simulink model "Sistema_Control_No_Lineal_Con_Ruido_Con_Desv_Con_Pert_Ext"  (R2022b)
settings: Solver=ode4  StartTime=0.0  StopTime=0.7  FixedStep=1e-6  RelTol=1e-3
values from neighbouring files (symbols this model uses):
  C_DC = 6.8e-3    (= 0.0068)    [Sistema_control_no_lineal_LQR.m]    (also in Sistema_control_no_lineal_Modal.m; PI_Lazo_V_DC.m; LQR_Sin_Integral.m; LQR_Con_Integral.m)
  control = eye(2)    [Sistema_control_no_lineal_LQR.m]    (also in Sistema_control_no_lineal_Modal.m; Sistema_no_lineal_Modal.m; Sistema_no_lineal_LQR.m)
  eta_d0_1 = ((i_q0_1*omega_1 + v_d_1/L_1 - (R_1/L_1)*i_d0_1)*(2*m_t1*L_1))/V_DC0    [Sistema_control_no_lineal_LQR.m]    (also in Sistema_control_no_lineal_Modal.m; Sistema_no_lineal_Modal.m; Sistema_no_lineal_LQR.m)
  eta_d0_2 = ((i_q0_2*omega_2 + v_d_2/L_2 - (R_2/L_2)*i_d0_2)*(2*m_t2*L_2))/V_DC0    [Sistema_control_no_lineal_LQR.m]    (also in Sistema_control_no_lineal_Modal.m; Sistema_no_lineal_Modal.m; Sistema_no_lineal_LQR.m)
  eta_q0_1 = (- i_d0_1*omega_1 - (R_1/L_1)*i_q0_1)*(2*m_t1*L_1)/V_DC0    [Sistema_control_no_lineal_LQR.m]    (also in Sistema_control_no_lineal_Modal.m; Sistema_no_lineal_Modal.m; Sistema_no_lineal_LQR.m)
  eta_q0_2 = ((- i_d0_2*omega_2 - (R_2/L_2)*i_q0_2)*(2*m_t2*L_2))/V_DC0    [Sistema_control_no_lineal_LQR.m]    (also in Sistema_control_no_lineal_Modal.m; Sistema_no_lineal_Modal.m; Sistema_no_lineal_LQR.m)
  i_d0_1 = ((3000*2)/(3*v_d_1))*1.06522    [Sistema_control_no_lineal_LQR.m]    (also in Sistema_control_no_lineal_Modal.m; PI_Lazo_V_DC.m = 14.14213562; Sistema_no_lineal_Modal.m; Sistema_no_lineal_LQR.m)
  i_d0_2 = -i_d0_1/1.06522    [Sistema_control_no_lineal_LQR.m]    (also in Sistema_control_no_lineal_Modal.m; Sistema_no_lineal_Modal.m; Sistema_no_lineal_LQR.m)
  I_p_i_d_1 = 0.2    [Sistema_control_no_lineal_LQR.m]    (also in Sistema_control_no_lineal_Modal.m; Sistema_no_lineal_Modal.m = 0.02; Sistema_no_lineal_LQR.m = 0.02)
  I_p_i_d_2 = 0.2    [Sistema_control_no_lineal_LQR.m]    (also in Sistema_control_no_lineal_Modal.m; Sistema_no_lineal_Modal.m = 0.02; Sistema_no_lineal_LQR.m = 0.02)
  I_p_i_q_1 = 0.2    [Sistema_control_no_lineal_LQR.m]    (also in Sistema_control_no_lineal_Modal.m; Sistema_no_lineal_Modal.m = 0.02; Sistema_no_lineal_LQR.m = 0.02)
  i_q0_1 = 0    [Sistema_control_no_lineal_LQR.m]    (also in Sistema_control_no_lineal_Modal.m; Sistema_no_lineal_Modal.m; Sistema_no_lineal_LQR.m)
  i_q0_2 = 0    [Sistema_control_no_lineal_LQR.m]    (also in Sistema_control_no_lineal_Modal.m; Sistema_no_lineal_Modal.m; Sistema_no_lineal_LQR.m)
  Inst_Desv_C_DC = 0.1    [Sistema_control_no_lineal_LQR.m]    (also in Sistema_control_no_lineal_Modal.m; Sistema_no_lineal_Modal.m; Sistema_no_lineal_LQR.m)
  Inst_Desv_L_1 = 0.1    [Sistema_control_no_lineal_LQR.m]    (also in Sistema_control_no_lineal_Modal.m; Sistema_no_lineal_Modal.m; Sistema_no_lineal_LQR.m)
  Inst_Desv_L_2 = 0.1    [Sistema_control_no_lineal_LQR.m]    (also in Sistema_control_no_lineal_Modal.m; Sistema_no_lineal_Modal.m; Sistema_no_lineal_LQR.m)
  Inst_Desv_R_1 = 0.1    [Sistema_control_no_lineal_LQR.m]    (also in Sistema_control_no_lineal_Modal.m; Sistema_no_lineal_Modal.m; Sistema_no_lineal_LQR.m)
  Inst_Desv_R_2 = 0.1    [Sistema_control_no_lineal_LQR.m]    (also in Sistema_control_no_lineal_Modal.m; Sistema_no_lineal_Modal.m; Sistema_no_lineal_LQR.m)
  Kc1 = Kca1(:, 1:2)    [Sistema_control_no_lineal_LQR.m]    (also in Sistema_control_no_lineal_Modal.m = Kca_place1(:, 1:2); Sistema_no_lineal_Modal.m = Kca_place1(:, 1:2); Sistema_no_lineal_LQR.m)
  Kc2 = Kca2(:, 1:2)    [Sistema_control_no_lineal_LQR.m]    (also in Sistema_control_no_lineal_Modal.m = Kca_place2(:, 1:2); Sistema_no_lineal_Modal.m = Kca_place2(:, 1:2); Sistema_no_lineal_LQR.m)
  Ki1 = -Kca1(:, 3:4)    [Sistema_control_no_lineal_LQR.m]    (also in Sistema_control_no_lineal_Modal.m = -Kca_place1(:, 3:4); Sistema_no_lineal_Modal.m = -Kca_place1(:, 3:4); Sistema_no_lineal_LQR.m)
  Ki2 = -Kca2(:, 3:4)    [Sistema_control_no_lineal_LQR.m]    (also in Sistema_control_no_lineal_Modal.m = -Kca_place2(:, 3:4); Sistema_no_lineal_Modal.m = -Kca_place2(:, 3:4); Sistema_no_lineal_LQR.m)
  Ki_DC = q_12/q_22    [Sistema_control_no_lineal_LQR.m]    (also in Sistema_control_no_lineal_Modal.m; PI_Lazo_V_DC.m)
  Ki_P = ((2+3*v_d_2*Kp_P)/(3*v_d_2*tau_P))    [Sistema_control_no_lineal_LQR.m]    (also in Sistema_control_no_lineal_Modal.m; IP_Lazo_P_2.m = ((2+3*v_d_2*Kp_P)/(3*v_d_2*tau)))
  Ki_Q = ((3*v_d_1*Kp_Q-2)/(3*v_d_1*tau_Q))    [Sistema_control_no_lineal_LQR.m]    (also in Sistema_control_no_lineal_Modal.m; IP_Lazo_Q_12.m = ((3*v_d_12*Kp_Q-2)/(3*v_d_12*tau)))
  Kp_DC = q_11/q_21    [Sistema_control_no_lineal_LQR.m]    (also in Sistema_control_no_lineal_Modal.m; PI_Lazo_V_DC.m)
  Kp_P = 0.0002    [Sistema_control_no_lineal_LQR.m]    (also in Sistema_control_no_lineal_Modal.m; IP_Lazo_P_2.m = 1)
  Kp_Q = 0.0002    [Sistema_control_no_lineal_LQR.m]    (also in Sistema_control_no_lineal_Modal.m; IP_Lazo_Q_12.m = 1)
  L_1 = 4.1e-3    (= 0.0041)    [Sistema_control_no_lineal_LQR.m]    (also in Sistema_control_no_lineal_Modal.m; Generadores_y_tranformadas.m; LQR_Sin_Integral.m; LQR_Con_Integral.m)
  L_2 = 5.3e-3    (= 0.0053)    [Sistema_control_no_lineal_LQR.m]    (also in Sistema_control_no_lineal_Modal.m; Generadores_y_tranformadas.m; Sistema_no_lineal_Modal.m; Sistema_no_lineal_LQR.m)
  lim_i_d_1_lower = -75.07117    [Sistema_control_no_lineal_LQR.m]    (also in Sistema_control_no_lineal_Modal.m; PI_Lazo_V_DC.m)
  lim_i_d_1_upper = 75.07117    [Sistema_control_no_lineal_LQR.m]    (also in Sistema_control_no_lineal_Modal.m; PI_Lazo_V_DC.m)
  lim_i_d_2_lower = -75.07117    [Sistema_control_no_lineal_LQR.m]    (also in Sistema_control_no_lineal_Modal.m; IP_Lazo_P_2.m)
  lim_i_d_2_upper = 75.07117    [Sistema_control_no_lineal_LQR.m]    (also in Sistema_control_no_lineal_Modal.m; IP_Lazo_P_2.m)
  lim_i_q_1_lower = -576.70686    [Sistema_control_no_lineal_LQR.m]    (also in Sistema_control_no_lineal_Modal.m; IP_Lazo_Q_12.m)
  lim_i_q_1_upper = 393.72177    [Sistema_control_no_lineal_LQR.m]    (also in Sistema_control_no_lineal_Modal.m; IP_Lazo_Q_12.m)
  m_t1 = 5    [Sistema_control_no_lineal_LQR.m]    (also in Sistema_control_no_lineal_Modal.m; LQR_Sin_Integral.m; LQR_Con_Integral.m; Modal_Integral.m)
  m_t2 = 5    [Sistema_control_no_lineal_LQR.m]    (also in Sistema_control_no_lineal_Modal.m; Sistema_no_lineal_Modal.m; Sistema_no_lineal_LQR.m)
  omega_1 = 377    [Sistema_control_no_lineal_LQR.m]    (also in Sistema_control_no_lineal_Modal.m; LQR_Sin_Integral.m; LQR_Con_Integral.m; Modal_Integral.m)
  omega_2 = 377    [Sistema_control_no_lineal_LQR.m]    (also in Sistema_control_no_lineal_Modal.m; Sistema_no_lineal_Modal.m; Sistema_no_lineal_LQR.m)
  P_2_1 = -3000    [Sistema_control_no_lineal_LQR.m]    (also in Sistema_control_no_lineal_Modal.m; IP_Lazo_P_2.m)
  P_2_2 = 3000    [Sistema_control_no_lineal_LQR.m]    (also in Sistema_control_no_lineal_Modal.m; IP_Lazo_P_2.m)
  P_2_3 = -8000    [Sistema_control_no_lineal_LQR.m]    (also in Sistema_control_no_lineal_Modal.m)
  p_i_d_1 = 2.5    [Sistema_control_no_lineal_LQR.m]    (also in Sistema_control_no_lineal_Modal.m; Sistema_no_lineal_Modal.m = 1.5; Sistema_no_lineal_LQR.m = 1.5)
  p_i_d_2 = 2.7    [Sistema_control_no_lineal_LQR.m]    (also in Sistema_control_no_lineal_Modal.m; Sistema_no_lineal_Modal.m = 1.7; Sistema_no_lineal_LQR.m = 1.7)
  p_i_q_1 = -0.5    [Sistema_control_no_lineal_LQR.m]    (also in Sistema_control_no_lineal_Modal.m; Sistema_no_lineal_Modal.m = -1.3; Sistema_no_lineal_LQR.m = -1.3)
  Porc_Desv_C_DC = 0.05    [Sistema_control_no_lineal_LQR.m]    (also in Sistema_control_no_lineal_Modal.m; Sistema_no_lineal_Modal.m; Sistema_no_lineal_LQR.m)
  Porc_Desv_L_1 = 0.05    [Sistema_control_no_lineal_LQR.m]    (also in Sistema_control_no_lineal_Modal.m; Sistema_no_lineal_Modal.m; Sistema_no_lineal_LQR.m)
  Porc_Desv_L_2 = 0.05    [Sistema_control_no_lineal_LQR.m]    (also in Sistema_control_no_lineal_Modal.m; Sistema_no_lineal_Modal.m; Sistema_no_lineal_LQR.m)
  Porc_Desv_R_1 = 0.05    [Sistema_control_no_lineal_LQR.m]    (also in Sistema_control_no_lineal_Modal.m; Sistema_no_lineal_Modal.m; Sistema_no_lineal_LQR.m)
  Porc_Desv_R_2 = 0.05    [Sistema_control_no_lineal_LQR.m]    (also in Sistema_control_no_lineal_Modal.m; Sistema_no_lineal_Modal.m; Sistema_no_lineal_LQR.m)
  Q_1_1 = 0    [Sistema_control_no_lineal_LQR.m]    (also in Sistema_control_no_lineal_Modal.m; IP_Lazo_Q_12.m)
  Q_1_2 = 0    [Sistema_control_no_lineal_LQR.m]    (also in Sistema_control_no_lineal_Modal.m; IP_Lazo_Q_12.m = -2500)
  Q_1_3 = 0    [Sistema_control_no_lineal_LQR.m]    (also in Sistema_control_no_lineal_Modal.m)
  Q_2_1 = 0    [Sistema_control_no_lineal_LQR.m]    (also in Sistema_control_no_lineal_Modal.m; IP_Lazo_Q_12.m = -3000)
  Q_2_2 = 0    [Sistema_control_no_lineal_LQR.m]    (also in Sistema_control_no_lineal_Modal.m; IP_Lazo_Q_12.m = 1000)
  Q_2_3 = 0    [Sistema_control_no_lineal_LQR.m]    (also in Sistema_control_no_lineal_Modal.m)
  R_1 = 284e-3    (= 0.284)    [Sistema_control_no_lineal_LQR.m]    (also in Sistema_control_no_lineal_Modal.m; Generadores_y_tranformadas.m; LQR_Sin_Integral.m; LQR_Con_Integral.m)
  R_2 = 330e-3    (= 0.33)    [Sistema_control_no_lineal_LQR.m]    (also in Sistema_control_no_lineal_Modal.m; Generadores_y_tranformadas.m; Sistema_no_lineal_Modal.m; Sistema_no_lineal_LQR.m)
  v_d_1 = 100*sqrt(2)    [Sistema_control_no_lineal_LQR.m]    (also in Sistema_control_no_lineal_Modal.m; PI_Lazo_V_DC.m; LQR_Sin_Integral.m; LQR_Con_Integral.m)
  v_d_2 = 100*sqrt(2)    [Sistema_control_no_lineal_LQR.m]    (also in Sistema_control_no_lineal_Modal.m; IP_Lazo_P_2.m; Sistema_no_lineal_Modal.m; Sistema_no_lineal_LQR.m)
  V_DC0 = 500    [Sistema_control_no_lineal_LQR.m]    (also in Sistema_control_no_lineal_Modal.m; PI_Lazo_V_DC.m; LQR_Sin_Integral.m; LQR_Con_Integral.m)
  V_R_C = D_R_V^2    (= 0.0009)    [Sistema_control_no_lineal_LQR.m]    (also in Sistema_control_no_lineal_Modal.m)
  V_R_i = D_R_i^2    (= 2.5e-05)    [Sistema_control_no_lineal_LQR.m]    (also in Sistema_control_no_lineal_Modal.m; LQR_Con_Integral.m; Modal_Integral.m; Sistema_no_lineal_Modal.m)
  V_R_V = D_R_V^2    (= 0.0009)    [Sistema_control_no_lineal_LQR.m]    (also in Sistema_control_no_lineal_Modal.m; PI_Lazo_V_DC.m; Sistema_no_lineal_Modal.m = 4e-06; Sistema_no_lineal_LQR.m = 4e-06)

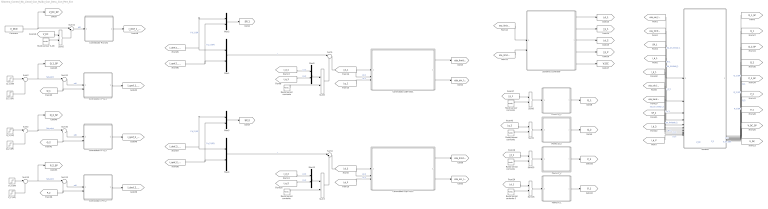
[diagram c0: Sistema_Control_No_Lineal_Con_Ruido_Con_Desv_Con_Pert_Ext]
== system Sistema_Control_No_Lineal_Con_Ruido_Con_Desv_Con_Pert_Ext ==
  "   Ruido sensor corriente " : RandomNumber  Variance=V_R_i  SampleTime=0.001
  "   Ruido sensor corriente 1" : RandomNumber  Variance=V_R_i  SampleTime=0.001
  "  Ruido sensor corriente " : RandomNumber  Variance=V_R_i  SampleTime=0.001
  " Ruido sensor corriente " : RandomNumber  Variance=V_R_i  SampleTime=0.001
  Constant : Constant  Value=V_DC0
  Controlador I-P P_2 : Subsystem
  Controlador I-P Q_1 : Subsystem
  Controlador I-P Q_2 : Subsystem
  Controlador LQR VSC1 : Subsystem
  Controlador LQR VSC2 : Subsystem
  Controlador PI V_DC : Subsystem
  Mux{1..2,4..5,9,12} (6 alike) : Mux  Inputs=2
  P_2 (SP) : Step  Time=0.3  Before=P_2_1  After=P_2_2  SampleTime=0
  "P_2 (SP) " : Step  Time=0.5  After=P_2_3  SampleTime=0
  Planta P_1 : Subsystem
  Planta P_2 : Subsystem
  Planta Q_1 : Subsystem
  Planta Q_2 : Subsystem
  Q_1 (SP) : Step  Time=0.3  Before=Q_1_1  After=Q_1_2  SampleTime=0
  "Q_1 (SP) " : Step  Time=0.5  After=Q_1_3  SampleTime=0
  Q_2 (SP) : Step  Time=0.4  Before=Q_2_1  After=Q_2_2  SampleTime=0
  "Q_2 (SP) " : Step  Time=0.5  After=Q_2_3  SampleTime=0
  Ruido sensor V_DC : RandomNumber  Variance=V_R_V  SampleTime=0.001
  Ruido sensor corriente : RandomNumber  Variance=V_R_i  SampleTime=0.001
  "Ruido sensor corriente " : RandomNumber  Variance=V_R_i  SampleTime=0.001
  Señales : Subsystem
  Sistema a controlar : Subsystem
  Sum{1,4,10..13} (6 alike) : Sum  Inputs=|+-
  Sum14 : Sum  Inputs=|++
  Sum{5..9,15..16} (7 alike) : Sum
  Sum2 : Sum  Inputs=|++
  Sum3 : Sum  Inputs=|++
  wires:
  Mux2/1 -> [SP_1]
  [i_dref_1_limitado] -> Mux2/1, Mux1/1  "i^d_1 (SP)"
  [i_qref_1_limitado] -> Mux2/2, Mux1/2  "i^q_1 (SP)"
  Mux1/1 -> Sum1/1  "r"
  [i_qref_2_limitado] -> Mux5/2, Mux4/2  "i^q_2 (SP)"
  [i_dref_2_limitado] -> Mux4/1, Mux5/1  "i^d_2 (SP)"
  Mux5/1 -> [SP_2]
  Sistema a controlar/1(i_d_1) -> [i_d_1]
  Sistema a controlar/2(i_q_1) -> [i_q_1]
  Sistema a controlar/3(i_d_2) -> [i_d_2]
  Sistema a controlar/4(i_q_2) -> [i_q_2]
  Sistema a controlar/5(V_DC) -> [V_DC]
  [eta_limitado_1] -> Sistema a controlar/1(eta limitado 1)
  [eta_limitado_2] -> Sistema a controlar/2(eta limitado 2)
  [i_d_1] -> Mux9/1  "i_d_2"
  [i_q_1] -> Mux9/2  "i_q_2"
  Sum6/1 -> Sum1/2
  Sum7/1 -> Sum4/2
  [i_q_2] -> Mux12/2  "i_q_2"
  [i_d_2] -> Mux12/1  "i_d_2"
  Mux4/1 -> Sum4/1  "r"
  Sum1/1 -> Controlador LQR VSC1/1(e)
  [i_d_1] -> Controlador LQR VSC1/2(i_d_1)  "i_d_1"
  [i_q_1] -> Controlador LQR VSC1/3(i_q_1)  "i_q_1"
  Controlador LQR VSC1/1(eta limitado 1) -> [eta_limitado_1]
  Controlador LQR VSC1/2(eta sin limitar 1) -> [eta_sin_limitar_1]
  Sum4/1 -> Controlador LQR VSC2/1(e)
  [i_d_2] -> Controlador LQR VSC2/2(i_d_2)  "i_d_2"
  [i_q_2] -> Controlador LQR VSC2/3(i_q_2)  "i_q_2"
  Controlador LQR VSC2/1(eta limitado 2) -> [eta_limitado_2]
  Controlador LQR VSC2/2(eta sin limitar 2) -> [eta_sin_limitar_2]
  Controlador I-P Q_1/1(i^q*_1 limitado) -> [i_qref_1_limitado]
  Sum12/1 -> Controlador I-P Q_1/1(e(t))  "e(t)"
  P_2 (SP)/1 -> Sum14/1
  Sum3/1 -> [Q_1_SP], Sum12/1  "Set-point"
  Controlador PI V_DC/1(i^d*_1 limitado) -> [i_dref_1_limitado]
  Sum13/1 -> Controlador I-P P_2/1(e(t))  "e(t)"
  Sum11/1 -> Controlador PI V_DC/1(e(t))  "e(t)"
  "P_2 (SP) "/1 -> Sum14/2
  Sum5/1 -> Sum11/2
  Controlador I-P P_2/1(i^d*_2 limitado) -> [i_dref_2_limitado]
  Sum10/1 -> Controlador I-P Q_2/1(e(t))  "e(t)"
  [P_2] -> Controlador I-P P_2/2(P_2), Sum13/2
  [Q_1] -> Controlador I-P Q_1/2(Q_1), Sum12/2
  [Q_2] -> Sum10/2, Controlador I-P Q_2/2(Q_1)
  Controlador I-P Q_2/1(i^q*_1 limitado) -> [i_qref_2_limitado]
  Sum2/1 -> Sum10/1, [Q_2_SP]  "Set-point"
  Sum14/1 -> [P_2_SP], Sum13/1  "Set-point"
  Constant/1 -> [V_DC_SP], Sum11/1
  Q_2 (SP)/1 -> Sum2/1
  "Q_2 (SP) "/1 -> Sum2/2
  Q_1 (SP)/1 -> Sum3/1
  "Q_1 (SP) "/1 -> Sum3/2
  [V_DC] -> Sum5/1
  Ruido sensor V_DC/1 -> Sum5/2
  Mux9/1 -> Sum6/1
  Ruido sensor corriente/1 -> Sum6/2
  Mux12/1 -> Sum7/1
  "Ruido sensor corriente "/1 -> Sum7/2
  [V_DC_SP] -> Señales/18(V_DC (SP))  "V_DC (SP)"
  [eta_limitado_1] -> Señales/2(eta_limitado_1)  "eta_limitado_1"
  [P_2] -> Señales/16(P_2)  "P_2"
  [i_q_1] -> Señales/5(i_q_1)  "i_q_1"
  [i_d_2] -> Señales/9(i_d_2)  "i_d_1"
  [i_q_2] -> Señales/10(i_q_2)  "i_q_1"
  [eta_sin_limitar_2] -> Señales/6(eta_sin_limitar_2)  "eta_sin_limitar_2"
  [Q_1] -> Señales/12(Q_1)  "Q_1"
  [eta_sin_limitar_1] -> Señales/1(eta_sin_limitar_1)  "eta_sin_limitar_1"
  [SP_2] -> Señales/8(SP_2)  "SP_2"
  [Q_1_SP] -> Señales/11(Q_1 (SP))  "Q_1 (SP)"
  [eta_limitado_2] -> Señales/7(eta_limitado_2)  "eta_limitado_2"
  [i_d_1] -> Señales/4(i_d_1)  "i_d_1"
  [P_2_SP] -> Señales/15(P_2 (SP))  "P_2 (SP)"
  [Q_2_SP] -> Señales/13(Q_2 (SP))  "Q_2 (SP)"
  [SP_1] -> Señales/3(SP_1)  "SP_1"
  [Q_2] -> Señales/14(Q_2)  "Q_2"
  [P_1] -> Señales/17(P_1)  "P_1"
  [V_DC] -> Señales/19(V_DC)  "V_DC"
  [i_q_2] -> Sum9/1
  Planta P_2/1(P_2) -> [P_2]
  [i_d_2] -> Sum15/1
  Planta Q_2/1(Q_2) -> [Q_2]
  "  Ruido sensor corriente "/1 -> Sum9/2
  [i_d_1] -> Sum16/1
  Sum16/1 -> Planta P_1/1(i^d*_1 limitado)
  Planta P_1/1(P_1) -> [P_1]
  Planta Q_1/1(Q_1) -> [Q_1]
  [i_q_1] -> Sum8/1
  " Ruido sensor corriente "/1 -> Sum8/2
  Sum8/1 -> Planta Q_1/1(i^q*_1 limitado)
  "   Ruido sensor corriente "/1 -> Sum15/2
  Sum9/1 -> Planta Q_2/1(i^q*_2 limitado)
  Sum15/1 -> Planta P_2/1(i^d*_2 limitado)
  "   Ruido sensor corriente 1"/1 -> Sum16/2

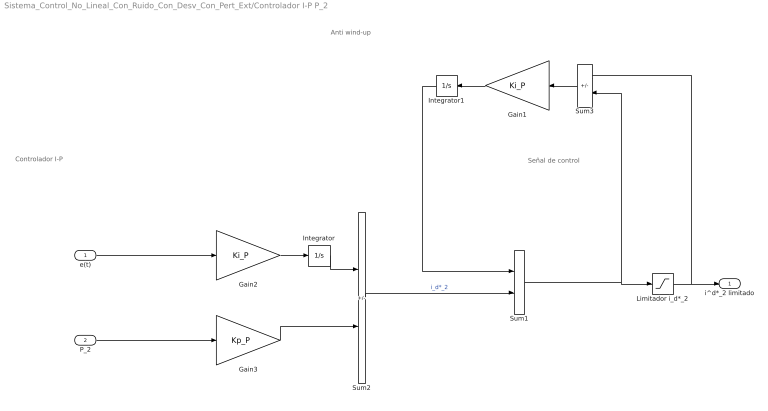
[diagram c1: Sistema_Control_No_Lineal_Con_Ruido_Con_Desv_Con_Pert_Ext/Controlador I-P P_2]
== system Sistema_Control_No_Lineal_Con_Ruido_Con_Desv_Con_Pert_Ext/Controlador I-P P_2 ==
  note: Señal de control
  note: Controlador I-P
  note: Anti wind-up
  e(t) : Inport
  P_2 : Inport  Port=2
  Gain1 : Gain  Gain=Ki_P
  Gain2 : Gain  Gain=Ki_P
  Gain3 : Gain  Gain=Kp_P
  Integrator : Integrator
  Integrator1 : Integrator
  Limitador i_d*_2 : Saturate  UpperLimit=lim_i_d_2_upper  LowerLimit=lim_i_d_2_lower
  Sum1 : Sum
  Sum2 : Sum  Inputs=+-
  Sum3 : Sum  Inputs=+-
  i^d*_2 limitado : Outport
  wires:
  Limitador i_d*_2/1 -> i^d*_2 limitado/1, Sum3/1
  Sum1/1 -> Limitador i_d*_2/1, Sum3/2
  Sum2/1 -> Sum1/2  "i_d*_2"
  Gain2/1 -> Integrator/1
  Integrator/1 -> Sum2/1
  e(t)/1 -> Gain2/1
  Sum3/1 -> Gain1/1
  Gain1/1 -> Integrator1/1
  Integrator1/1 -> Sum1/1
  P_2/1 -> Gain3/1
  Gain3/1 -> Sum2/2

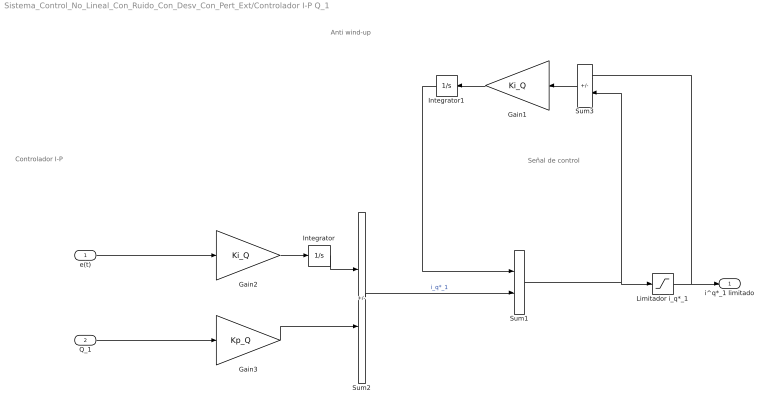
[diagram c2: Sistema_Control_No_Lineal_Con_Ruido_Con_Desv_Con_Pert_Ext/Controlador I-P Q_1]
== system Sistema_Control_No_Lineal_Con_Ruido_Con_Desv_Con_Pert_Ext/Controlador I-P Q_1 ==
  note: Señal de control
  note: Controlador I-P
  note: Anti wind-up
  e(t) : Inport
  Q_1 : Inport  Port=2
  Gain1 : Gain  Gain=Ki_Q
  Gain2 : Gain  Gain=Ki_Q
  Gain3 : Gain  Gain=Kp_Q
  Integrator : Integrator
  Integrator1 : Integrator
  Limitador i_q*_1 : Saturate  UpperLimit=lim_i_q_1_upper  LowerLimit=lim_i_q_1_lower
  Sum1 : Sum
  Sum2 : Sum  Inputs=+-
  Sum3 : Sum  Inputs=+-
  i^q*_1 limitado : Outport
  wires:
  Limitador i_q*_1/1 -> i^q*_1 limitado/1, Sum3/1
  Sum1/1 -> Limitador i_q*_1/1, Sum3/2
  Sum2/1 -> Sum1/2  "i_q*_1"
  Gain2/1 -> Integrator/1
  Integrator/1 -> Sum2/1
  e(t)/1 -> Gain2/1
  Sum3/1 -> Gain1/1
  Gain1/1 -> Integrator1/1
  Integrator1/1 -> Sum1/1
  Q_1/1 -> Gain3/1
  Gain3/1 -> Sum2/2

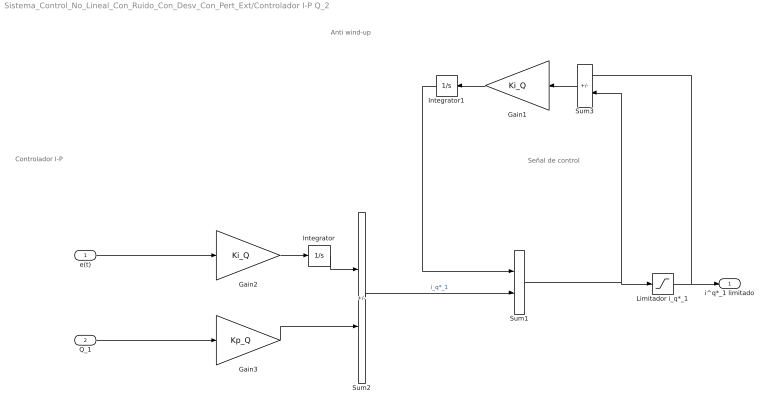
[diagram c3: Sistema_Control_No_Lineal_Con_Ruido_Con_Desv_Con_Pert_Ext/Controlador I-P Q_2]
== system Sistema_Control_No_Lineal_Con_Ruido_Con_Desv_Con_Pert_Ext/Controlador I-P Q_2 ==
  note: Anti wind-up
  note: Controlador I-P
  note: Señal de control
  e(t) : Inport
  Q_1 : Inport  Port=2
  Gain1 : Gain  Gain=Ki_Q
  Gain2 : Gain  Gain=Ki_Q
  Gain3 : Gain  Gain=Kp_Q
  Integrator : Integrator
  Integrator1 : Integrator
  Limitador i_q*_1 : Saturate  UpperLimit=lim_i_q_1_upper  LowerLimit=lim_i_q_1_lower
  Sum1 : Sum
  Sum2 : Sum  Inputs=+-
  Sum3 : Sum  Inputs=+-
  i^q*_1 limitado : Outport
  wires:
  Gain3/1 -> Sum2/2
  Q_1/1 -> Gain3/1
  Integrator1/1 -> Sum1/1
  Gain1/1 -> Integrator1/1
  Sum3/1 -> Gain1/1
  e(t)/1 -> Gain2/1
  Integrator/1 -> Sum2/1
  Gain2/1 -> Integrator/1
  Sum2/1 -> Sum1/2  "i_q*_1"
  Sum1/1 -> Sum3/2, Limitador i_q*_1/1
  Limitador i_q*_1/1 -> Sum3/1, i^q*_1 limitado/1

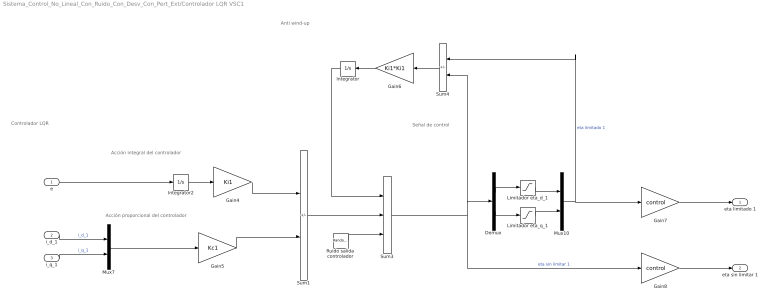
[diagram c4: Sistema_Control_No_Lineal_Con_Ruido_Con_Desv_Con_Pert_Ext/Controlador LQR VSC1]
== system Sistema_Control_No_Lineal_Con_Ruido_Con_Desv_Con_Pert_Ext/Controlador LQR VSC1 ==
  note: Anti wind-up
  note: Controlador LQR
  note: Acción proporcional del controlador
  note: Acción integral del controlador
  note: Señal de control
  e : Inport
  i_d_1 : Inport  Port=2
  i_q_1 : Inport  Port=3
  Demux : Demux  Outputs=2
  Gain4 : Gain  Gain=Ki1  Multiplication=Matrix(K*u) (u vector)
  Gain5 : Gain  Gain=Kc1  Multiplication=Matrix(K*u) (u vector)
  Gain6 : Gain  Gain=Ki1*Ki1  Multiplication=Matrix(K*u) (u vector)
  Gain7 : Gain  Gain=control  Multiplication=Matrix(K*u) (u vector)
  Gain8 : Gain  Gain=control  Multiplication=Matrix(K*u) (u vector)
  Integrator : Integrator
  Integrator2 : Integrator
  Limitador eta_d_1 : Saturate  UpperLimit=5 - eta_d0_1  LowerLimit=-5 - eta_d0_1
  Limitador eta_q_1 : Saturate  UpperLimit=5 - eta_q0_1  LowerLimit=-5 - eta_q0_1
  Mux10 : Mux  Inputs=2
  Mux7 : Mux  Inputs=2
  Ruido salida controlador : RandomNumber  Variance=V_R_C  SampleTime=0.001
  Sum1 : Sum  Inputs=+-
  Sum3 : Sum  Inputs=+++
  Sum4 : Sum  Inputs=+-
  eta limitado 1 : Outport
  eta sin limitar 1 : Outport  Port=2
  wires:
  i_q_1/1 -> Mux7/2  "i_q_1"
  Mux10/1 -> Sum4/1, Gain7/1  "eta limitado 1"
  Limitador eta_q_1/1 -> Mux10/2
  i_d_1/1 -> Mux7/1  "i_d_1"
  Limitador eta_d_1/1 -> Mux10/1
  Demux/2 -> Limitador eta_q_1/1
  Gain8/1 -> eta sin limitar 1/1
  Sum3/1 -> Demux/1, Sum4/2, Gain8/1  "eta sin limitar 1"
  Gain7/1 -> eta limitado 1/1
  Demux/1 -> Limitador eta_d_1/1
  Gain5/1 -> Sum1/2
  Gain4/1 -> Sum1/1
  Sum4/1 -> Gain6/1
  Mux7/1 -> Gain5/1
  Gain6/1 -> Integrator/1
  Sum1/1 -> Sum3/2
  Integrator2/1 -> Gain4/1
  e/1 -> Integrator2/1
  Integrator/1 -> Sum3/1
  Ruido salida controlador/1 -> Sum3/3

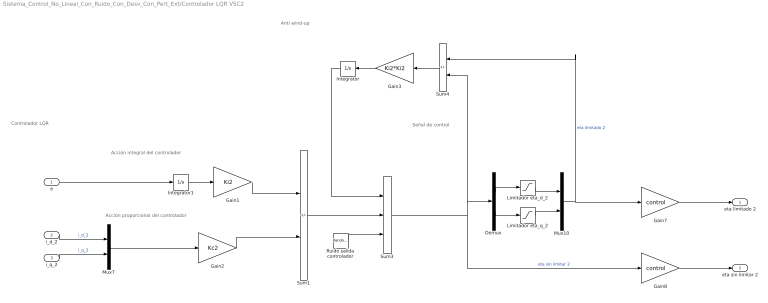
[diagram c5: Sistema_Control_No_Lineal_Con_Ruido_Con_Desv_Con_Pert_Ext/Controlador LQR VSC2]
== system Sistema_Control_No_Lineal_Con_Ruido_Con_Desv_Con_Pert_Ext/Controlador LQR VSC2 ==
  note: Señal de control
  note: Anti wind-up
  note: Acción proporcional del controlador
  note: Controlador LQR
  note: Acción integral del controlador
  e : Inport
  i_d_2 : Inport  Port=2
  i_q_2 : Inport  Port=3
  Demux : Demux  Outputs=2
  Gain1 : Gain  Gain=Ki2  Multiplication=Matrix(K*u) (u vector)
  Gain2 : Gain  Gain=Kc2  Multiplication=Matrix(K*u) (u vector)
  Gain3 : Gain  Gain=Ki2*Ki2  Multiplication=Matrix(K*u) (u vector)
  Gain7 : Gain  Gain=control  Multiplication=Matrix(K*u) (u vector)
  Gain8 : Gain  Gain=control  Multiplication=Matrix(K*u) (u vector)
  Integrator : Integrator
  Integrator1 : Integrator
  Limitador eta_d_2 : Saturate  UpperLimit=5 - eta_d0_2  LowerLimit=-5 - eta_d0_2
  Limitador eta_q_2 : Saturate  UpperLimit=5 - eta_q0_2  LowerLimit=-5 - eta_q0_2
  Mux10 : Mux  Inputs=2
  Mux7 : Mux  Inputs=2
  Ruido salida controlador : RandomNumber  Variance=V_R_C  SampleTime=0.001
  Sum1 : Sum  Inputs=+-
  Sum3 : Sum  Inputs=+++
  Sum4 : Sum  Inputs=+-
  eta limitado 2 : Outport
  eta sin limitar 2 : Outport  Port=2
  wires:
  Gain8/1 -> eta sin limitar 2/1
  Integrator/1 -> Sum3/1
  Mux7/1 -> Gain2/1
  i_d_2/1 -> Mux7/1  "i_d_2"
  Mux10/1 -> Sum4/1, Gain7/1  "eta limitado 2"
  Gain7/1 -> eta limitado 2/1
  Sum3/1 -> Demux/1, Sum4/2, Gain8/1  "eta sin limitar 2"
  i_q_2/1 -> Mux7/2  "i_q_2"
  Limitador eta_d_2/1 -> Mux10/1
  Limitador eta_q_2/1 -> Mux10/2
  Integrator1/1 -> Gain1/1
  Demux/2 -> Limitador eta_q_2/1
  Demux/1 -> Limitador eta_d_2/1
  Sum4/1 -> Gain3/1
  Gain3/1 -> Integrator/1
  Sum1/1 -> Sum3/2
  Gain1/1 -> Sum1/1
  Gain2/1 -> Sum1/2
  e/1 -> Integrator1/1
  Ruido salida controlador/1 -> Sum3/3

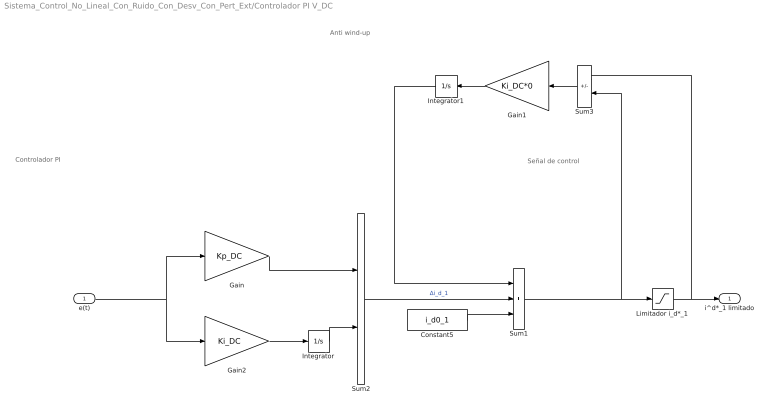
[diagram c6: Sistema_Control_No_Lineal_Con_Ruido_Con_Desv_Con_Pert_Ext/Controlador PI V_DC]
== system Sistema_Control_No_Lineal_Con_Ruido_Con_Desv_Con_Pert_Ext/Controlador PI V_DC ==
  note: Señal de control
  note: Controlador PI
  note: Anti wind-up
  e(t) : Inport
  Constant5 : Constant  Value=i_d0_1
  Gain : Gain  Gain=Kp_DC
  Gain1 : Gain  Gain=Ki_DC*0
  Gain2 : Gain  Gain=Ki_DC
  Integrator : Integrator
  Integrator1 : Integrator
  Limitador i_d*_1 : Saturate  UpperLimit=lim_i_d_1_upper  LowerLimit=lim_i_d_1_lower
  Sum1 : Sum  Inputs=+++
  Sum2 : Sum
  Sum3 : Sum  Inputs=+-
  i^d*_1 limitado : Outport
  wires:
  Limitador i_d*_1/1 -> Sum3/1, i^d*_1 limitado/1
  Constant5/1 -> Sum1/3
  Sum1/1 -> Sum3/2, Limitador i_d*_1/1
  Sum2/1 -> Sum1/2  "Δi_d_1"
  Gain2/1 -> Integrator/1
  Integrator/1 -> Sum2/2
  Gain/1 -> Sum2/1
  e(t)/1 -> Gain2/1, Gain/1
  Sum3/1 -> Gain1/1
  Gain1/1 -> Integrator1/1
  Integrator1/1 -> Sum1/1

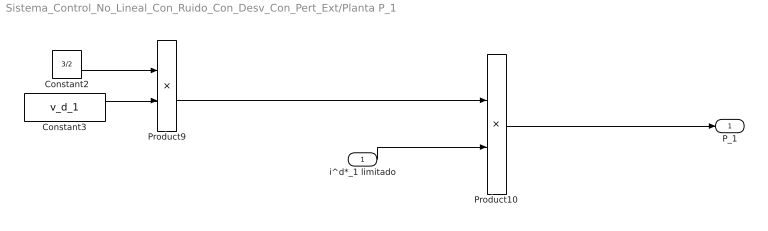
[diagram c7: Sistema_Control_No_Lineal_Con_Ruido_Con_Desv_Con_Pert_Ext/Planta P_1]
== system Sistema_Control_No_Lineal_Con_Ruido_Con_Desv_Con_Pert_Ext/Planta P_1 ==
  i^d*_1 limitado : Inport
  Constant2 : Constant  Value=3/2
  Constant3 : Constant  Value=v_d_1
  Product10 : Product
  Product9 : Product
  P_1 : Outport
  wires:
  Product10/1 -> P_1/1
  Constant2/1 -> Product9/1
  Constant3/1 -> Product9/2
  i^d*_1 limitado/1 -> Product10/2
  Product9/1 -> Product10/1

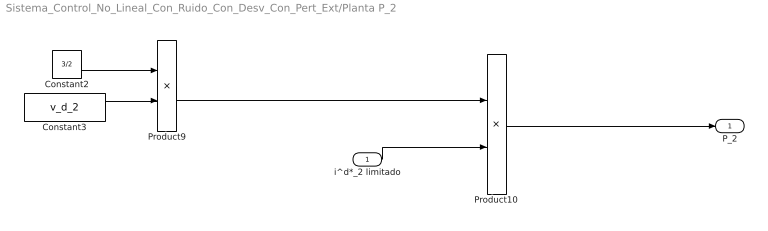
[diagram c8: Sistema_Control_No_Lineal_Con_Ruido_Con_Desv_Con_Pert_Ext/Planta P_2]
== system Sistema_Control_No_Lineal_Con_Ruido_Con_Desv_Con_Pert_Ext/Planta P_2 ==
  i^d*_2 limitado : Inport
  Constant2 : Constant  Value=3/2
  Constant3 : Constant  Value=v_d_2
  Product10 : Product
  Product9 : Product
  P_2 : Outport
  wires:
  Product9/1 -> Product10/1
  i^d*_2 limitado/1 -> Product10/2
  Constant3/1 -> Product9/2
  Constant2/1 -> Product9/1
  Product10/1 -> P_2/1

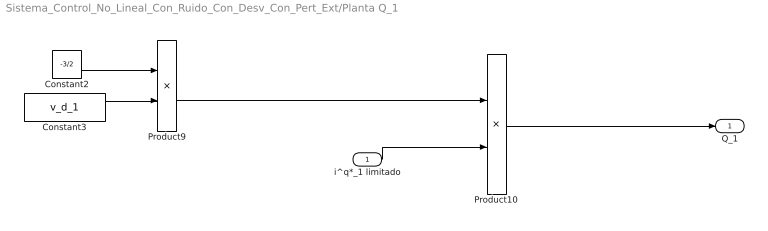
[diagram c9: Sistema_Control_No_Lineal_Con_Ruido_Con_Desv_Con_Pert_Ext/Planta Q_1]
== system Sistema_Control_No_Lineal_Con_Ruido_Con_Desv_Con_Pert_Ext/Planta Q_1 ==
  i^q*_1 limitado : Inport
  Constant2 : Constant  Value=-3/2
  Constant3 : Constant  Value=v_d_1
  Product10 : Product
  Product9 : Product
  Q_1 : Outport
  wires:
  Constant2/1 -> Product9/1
  Constant3/1 -> Product9/2
  i^q*_1 limitado/1 -> Product10/2
  Product9/1 -> Product10/1
  Product10/1 -> Q_1/1

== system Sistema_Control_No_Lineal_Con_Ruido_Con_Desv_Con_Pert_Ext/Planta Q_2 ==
  i^q*_2 limitado : Inport
  Constant2 : Constant  Value=-3/2
  Constant3 : Constant  Value=v_d_2
  Product10 : Product
  Product9 : Product
  Q_2 : Outport
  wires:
  Product9/1 -> Product10/1
  i^q*_2 limitado/1 -> Product10/2
  Constant3/1 -> Product9/2
  Constant2/1 -> Product9/1
  Product10/1 -> Q_2/1

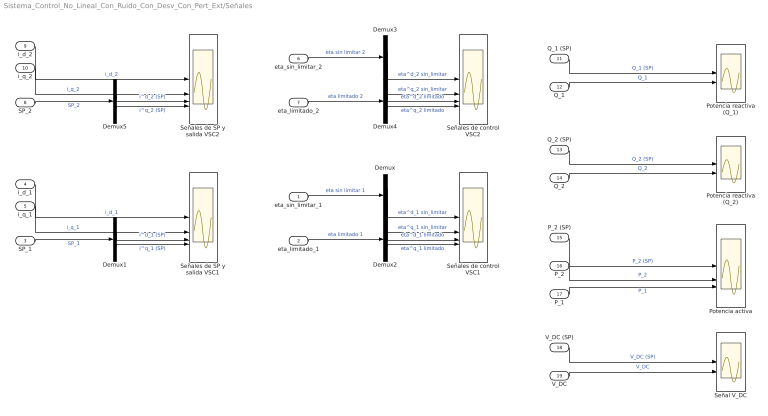
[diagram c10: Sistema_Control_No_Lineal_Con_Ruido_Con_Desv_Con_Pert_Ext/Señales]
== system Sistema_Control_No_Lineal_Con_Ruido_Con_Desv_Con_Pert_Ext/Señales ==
  eta_sin_limitar_1 : Inport
  eta_limitado_1 : Inport  Port=2
  SP_1 : Inport  Port=3
  i_d_1 : Inport  Port=4
  i_q_1 : Inport  Port=5
  eta_sin_limitar_2 : Inport  Port=6
  eta_limitado_2 : Inport  Port=7
  SP_2 : Inport  Port=8
  i_d_2 : Inport  Port=9
  i_q_2 : Inport  Port=10
  Q_1 (SP) : Inport  Port=11
  Q_1 : Inport  Port=12
  Q_2 (SP) : Inport  Port=13
  Q_2 : Inport  Port=14
  P_2 (SP) : Inport  Port=15
  P_2 : Inport  Port=16
  P_1 : Inport  Port=17
  V_DC (SP) : Inport  Port=18
  V_DC : Inport  Port=19
  Demux{,1..5} (6 alike) : Demux  Outputs=2
  Potencia activa : Scope  NumInputPorts=3
  Potencia reactiva (Q_1) : Scope  NumInputPorts=2
  Potencia reactiva (Q_2) : Scope  NumInputPorts=2
  Señal V_DC : Scope  NumInputPorts=2
  Señales de control VSC1 : Scope  NumInputPorts=4
  Señales de control VSC2 : Scope  NumInputPorts=4
  Señales de SP y salida VSC1 : Scope  NumInputPorts=4
  Señales de SP y salida VSC2 : Scope  NumInputPorts=4
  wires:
  i_d_1/1 -> Señales de SP y salida VSC1/1  "i_d_1"
  eta_sin_limitar_1/1 -> Demux/1  "eta sin limitar 1"
  SP_1/1 -> Demux1/1  "SP_1"
  eta_limitado_1/1 -> Demux2/1  "eta limitado 1"
  eta_sin_limitar_2/1 -> Demux3/1  "eta sin limitar 2"
  eta_limitado_2/1 -> Demux4/1  "eta limitado 2"
  SP_2/1 -> Demux5/1  "SP_2"
  i_q_1/1 -> Señales de SP y salida VSC1/2  "i_q_1"
  i_q_2/1 -> Señales de SP y salida VSC2/2  "i_q_2"
  i_d_2/1 -> Señales de SP y salida VSC2/1  "i_d_2"
  V_DC/1 -> Señal V_DC/2  "V_DC"
  Demux5/2 -> Señales de SP y salida VSC2/4  "i^q_2 (SP)"
  Demux5/1 -> Señales de SP y salida VSC2/3  "i^d_2 (SP)"
  Demux1/1 -> Señales de SP y salida VSC1/3  "i^d_1 (SP)"
  Demux1/2 -> Señales de SP y salida VSC1/4  "i^q_1 (SP)"
  Demux2/2 -> Señales de control VSC1/4  "eta^q_1 limitado"
  Demux/2 -> Señales de control VSC1/2  "eta^q_1 sin_limitar"
  Demux2/1 -> Señales de control VSC1/3  "eta^d_1 limitado"
  Demux/1 -> Señales de control VSC1/1  "eta^d_1 sin_limitar"
  Demux3/1 -> Señales de control VSC2/1  "eta^d_2 sin_limitar"
  Demux4/1 -> Señales de control VSC2/3  "eta^d_2 limitado"
  Demux3/2 -> Señales de control VSC2/2  "eta^q_2 sin_limitar"
  Demux4/2 -> Señales de control VSC2/4  "eta^q_2 limitado"
  Q_1 (SP)/1 -> Potencia reactiva (Q_1)/1  "Q_1 (SP)"
  Q_1/1 -> Potencia reactiva (Q_1)/2  "Q_1"
  Q_2 (SP)/1 -> Potencia reactiva (Q_2)/1  "Q_2 (SP)"
  Q_2/1 -> Potencia reactiva (Q_2)/2  "Q_2"
  P_2 (SP)/1 -> Potencia activa/1  "P_2 (SP)"
  P_2/1 -> Potencia activa/2  "P_2"
  V_DC (SP)/1 -> Señal V_DC/1  "V_DC (SP)"
  P_1/1 -> Potencia activa/3  "P_1"

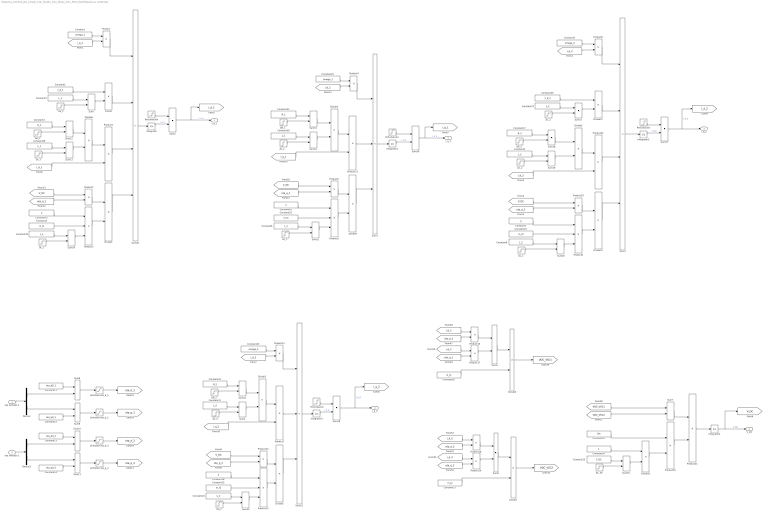
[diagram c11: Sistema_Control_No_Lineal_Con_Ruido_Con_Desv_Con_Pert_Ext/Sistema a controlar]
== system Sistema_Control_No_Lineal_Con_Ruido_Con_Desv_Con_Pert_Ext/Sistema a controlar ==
  eta limitado 1 : Inport
  eta limitado 2 : Inport  Port=2
  "  Perturbación " : Step  Time=I_p_i_d_2  After=p_i_d_2  SampleTime=0
  "  ΔL_2  " : Step  Time=Inst_Desv_L_2  After=L_2*Porc_Desv_L_2  SampleTime=0
  " Perturbación " : Step  Time=I_p_i_d_2  After=p_i_d_2  SampleTime=0
  " ΔL_1   " : Step  Time=Inst_Desv_L_1  After=L_1*Porc_Desv_L_1  SampleTime=0
  " ΔL_2  " : Step  Time=Inst_Desv_L_2  After=L_2*Porc_Desv_L_2  SampleTime=0
  Constant : Constant  Value=omega_1
  Constant1 : Constant  Value=v_d_1
  Constant11 : Constant  Value=eta_d0_1
  Constant12 : Constant  Value=eta_q0_1
  Constant13 : Constant  Value=eta_d0_2
  Constant14 : Constant  Value=eta_q0_2
  Constant{7,15..16,18} (4 alike) : Constant  Value=2
  Constant17 : Constant  Value=R_2
  Constant19 : Constant  Value=3/4
  Constant{2,8,28,30,36} (5 alike) : Constant  Value=L_1
  Constant20 : Constant  Value=omega_1
  Constant21 : Constant  Value=R_1
  Constant22 : Constant  Value=m_t1
  Constant23 : Constant  Value=omega_2
  Constant{6,9,24,31,37} (5 alike) : Constant  Value=L_2
  Constant25 : Constant  Value=m_t2
  Constant26 : Constant  Value=m_t1
  Constant27 : Constant  Value=m_t2
  Constant29 : Constant  Value=v_d_2
  Constant3 : Constant  Value=R_1
  Constant32 : Constant  Value=R_2
  Constant33 : Constant  Value=m_t2
  Constant34 : Constant
  Constant35 : Constant  Value=C_DC
  Constant4 : Constant  Value=m_t1
  Constant5 : Constant  Value=omega_2
  Demux : Demux  Outputs=2
  Demux1 : Demux  Outputs=2
  Divide{,1..12} (13 alike) : Product  Inputs=*/
  Integrator : Integrator  InitialCondition=i_d0_1
  Integrator1 : Integrator  InitialCondition=i_q0_1
  Integrator2 : Integrator  InitialCondition=i_d0_2
  Integrator3 : Integrator  InitialCondition=i_q0_2
  Integrator4 : Integrator  InitialCondition=V_DC0
  Limitador eta_d_1 : Saturate  UpperLimit=5  LowerLimit=-5
  Limitador eta_d_2 : Saturate  UpperLimit=5  LowerLimit=-5
  Limitador eta_q_1 : Saturate  UpperLimit=5  LowerLimit=-5
  Limitador eta_q_2 : Saturate  UpperLimit=5  LowerLimit=-5
  Perturbación : Step  Time=I_p_i_d_1  After=p_i_d_1  SampleTime=0
  "Perturbación " : Step  Time=I_p_i_q_1  After=p_i_q_1  SampleTime=0
  Product{,1..2,4,6..8,10..12,14,16..22} (18 alike) : Product
  Product{3,5,9,13} (4 alike) : Product  Inputs=3
  Sum{,2,4..21,23..25,27..28,30} (26 alike) : Sum
  Sum1 : Sum  Inputs=---
  Sum22 : Sum  Inputs=---
  Sum26 : Sum  Inputs=++--
  Sum3 : Sum  Inputs=++--
  ΔC_DC : Step  Time=Inst_Desv_C_DC  After=C_DC*Porc_Desv_C_DC  SampleTime=0
  ΔL_1 : Step  Time=Inst_Desv_L_1  After=L_1*Porc_Desv_L_1  SampleTime=0
  "ΔL_1 " : Step  Time=Inst_Desv_L_1  After=L_1*Porc_Desv_L_1  SampleTime=0
  "ΔL_1  " : Step  Time=Inst_Desv_L_1  After=L_1*Porc_Desv_L_1  SampleTime=0
  "ΔL_1   " : Step  Time=Inst_Desv_L_1  After=L_1*Porc_Desv_L_1  SampleTime=0
  ΔL_2 : Step  Time=Inst_Desv_L_2  After=L_2*Porc_Desv_L_2  SampleTime=0
  "ΔL_2 " : Step  Time=Inst_Desv_L_2  After=L_2*Porc_Desv_L_2  SampleTime=0
  "ΔL_2  " : Step  Time=Inst_Desv_L_2  After=L_2*Porc_Desv_L_2  SampleTime=0
  ΔR_1 : Step  Time=Inst_Desv_R_1  After=R_1*Porc_Desv_R_1  SampleTime=0
  "ΔR_1 " : Step  Time=Inst_Desv_R_1  After=R_1*Porc_Desv_R_1  SampleTime=0
  ΔR_2 : Step  Time=Inst_Desv_R_2  After=R_2*Porc_Desv_R_2  SampleTime=0
  "ΔR_2 " : Step  Time=Inst_Desv_R_2  After=R_2*Porc_Desv_R_2  SampleTime=0
  i_d_1 : Outport
  i_q_1 : Outport  Port=2
  i_d_2 : Outport  Port=3
  i_q_2 : Outport  Port=4
  V_DC : Outport  Port=5
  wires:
  Product21/1 -> Integrator4/1
  Product20/1 -> Product21/2
  Sum7/1 -> Product21/1
  Divide11/1 -> Product20/2
  Constant19/1 -> Product20/1
  [VDC_VSC2] -> Sum7/2
  [VDC_VSC1] -> Sum7/1
  Product18/1 -> Sum6/1
  Product19/1 -> Sum6/2
  [eta_d_2] -> Product18/2
  [eta_q_2] -> Product19/2
  [i_q_2] -> Product19/1
  [i_d_2] -> Product18/1
  Sum6/1 -> Divide7/1
  Constant27/1 -> Divide7/2
  Divide7/1 -> [VDC_VSC2]
  Divide6/1 -> [VDC_VSC1]
  Constant26/1 -> Divide6/2
  Sum5/1 -> Divide6/1
  [i_d_1] -> Product16/1
  [i_q_1] -> Product17/1
  [eta_q_1] -> Product17/2
  [eta_d_1] -> Product16/2
  Product17/1 -> Sum5/2
  Product16/1 -> Sum5/1
  Sum3/1 -> Integrator2/1
  Sum1/1 -> Integrator1/1
  [i_d_1] -> Product4/2
  Product4/1 -> Sum1/1
  Product11/1 -> Sum1/2
  [i_q_1] -> Product11/2
  Product6/1 -> Divide9/1
  Product5/1 -> Divide9/2
  Divide9/1 -> Sum1/3
  [V_DC] -> Product6/1
  [eta_q_1] -> Product6/2
  Constant16/1 -> Product5/1
  eta limitado 2/1 -> Demux1/1
  Constant15/1 -> Product3/1
  Constant4/1 -> Product3/2
  [eta_d_1] -> Product2/2
  [V_DC] -> Product2/1
  Divide1/1 -> Sum26/4
  Product3/1 -> Divide1/2
  Product2/1 -> Divide1/1
  [i_d_1] -> Product1/2
  Product1/1 -> Sum26/3
  Constant2/1 -> Sum/1
  Divide/1 -> Sum26/2
  Sum26/1 -> Integrator/1
  Product/1 -> Sum26/1
  [i_q_1] -> Product/2
  Integrator4/1 -> [V_DC], V_DC/1  "V_DC"
  Sum27/1 -> i_d_2/1, [i_d_2]  "i_d_2"
  Sum28/1 -> [i_q_2], i_q_2/1  "i_q_2"
  Sum30/1 -> i_q_1/1, [i_q_1]  "i_q_1"
  Constant/1 -> Product/1
  Sum2/1 -> i_d_1/1, [i_d_1]  "i_d_1"
  eta limitado 1/1 -> Demux/1
  Demux/1 -> Sum8/2
  Constant11/1 -> Sum8/1
  Sum8/1 -> Limitador eta_d_1/1
  Demux/2 -> Sum9/1
  Sum9/1 -> Limitador eta_q_1/1
  Constant12/1 -> Sum9/2
  Constant14/1 -> Sum11/2
  Demux1/2 -> Sum11/1
  Constant13/1 -> Sum10/1
  Demux1/1 -> Sum10/2
  Sum10/1 -> Limitador eta_d_2/1
  Sum11/1 -> Limitador eta_q_2/1
  Constant1/1 -> Divide/1
  Constant20/1 -> Product4/1
  Constant22/1 -> Product5/2
  Limitador eta_d_1/1 -> [eta_d_1]
  Limitador eta_q_1/1 -> [eta_q_1]
  Limitador eta_d_2/1 -> [eta_d_2]
  Limitador eta_q_2/1 -> [eta_q_2]
  Constant3/1 -> Sum12/1
  Constant28/1 -> Sum13/1
  Divide8/1 -> Product1/1
  Sum16/1 -> Divide4/2
  Constant21/1 -> Sum15/1
  Divide4/1 -> Product11/1
  Constant30/1 -> Sum14/1
  Sum21/1 -> Product5/3
  Sum20/1 -> Product9/3
  Divide2/1 -> Product22/1
  Constant9/1 -> Sum19/1
  Constant17/1 -> Sum18/1
  Constant5/1 -> Product8/1
  [i_q_2] -> Product8/2
  [i_d_2] -> Product22/2
  Product10/1 -> Divide10/1
  Product9/1 -> Divide10/2
  [V_DC] -> Product10/1
  [eta_d_2] -> Product10/2
  Constant33/1 -> Product9/2
  Constant7/1 -> Product9/1
  Product8/1 -> Sum3/1
  Divide12/1 -> Sum3/2
  Divide10/1 -> Sum3/4
  Product22/1 -> Sum3/3
  Sum24/1 -> Product13/3
  Sum23/1 -> Divide3/1
  Sum4/1 -> Divide3/2
  Constant25/1 -> Product13/2
  Constant23/1 -> Product12/1
  Constant18/1 -> Product13/1
  [eta_q_2] -> Product14/2
  [V_DC] -> Product14/1
  Divide5/1 -> Sum22/3
  Product13/1 -> Divide5/2
  Product14/1 -> Divide5/1
  [i_q_2] -> Product7/2
  Product7/1 -> Sum22/2
  Product12/1 -> Sum22/1
  [i_d_2] -> Product12/2
  ΔL_1/1 -> Sum/2
  Sum/1 -> Divide/2
  ΔR_1/1 -> Sum12/2
  "ΔL_1 "/1 -> Sum13/2
  Sum13/1 -> Divide8/2
  Sum12/1 -> Divide8/1
  "ΔL_1  "/1 -> Sum14/2
  Sum14/1 -> Product3/3
  "ΔR_1 "/1 -> Sum15/2
  Sum15/1 -> Divide4/1
  "ΔL_1   "/1 -> Sum16/2
  Constant36/1 -> Sum16/1
  ΔL_2/1 -> Sum17/2
  Sum17/1 -> Divide12/2
  Constant37/1 -> Sum17/1
  Constant29/1 -> Divide12/1
  Sum18/1 -> Divide2/1
  Sum19/1 -> Divide2/2
  "ΔL_2 "/1 -> Sum19/2
  ΔR_2/1 -> Sum18/2
  "ΔL_2  "/1 -> Sum20/2
  Constant6/1 -> Sum20/1
  Constant8/1 -> Sum21/1
  " ΔL_1   "/1 -> Sum21/2
  Divide3/1 -> Product7/1
  Constant31/1 -> Sum4/1
  " ΔL_2  "/1 -> Sum4/2
  "ΔR_2 "/1 -> Sum23/2
  Constant32/1 -> Sum23/1
  "  ΔL_2  "/1 -> Sum24/2
  Constant24/1 -> Sum24/1
  Constant34/1 -> Divide11/1
  Constant35/1 -> Sum25/1
  ΔC_DC/1 -> Sum25/2
  Sum25/1 -> Divide11/2
  Perturbación/1 -> Sum2/1
  " Perturbación "/1 -> Sum27/1
  "  Perturbación "/1 -> Sum28/1
  Sum22/1 -> Integrator3/1
  Integrator/1 -> Sum2/2  "i_d_1"
  Integrator1/1 -> Sum30/2  "i_q_1"
  "Perturbación "/1 -> Sum30/1
  Integrator2/1 -> Sum27/2  "i_d_2"
  Integrator3/1 -> Sum28/2  "i_q_2"
